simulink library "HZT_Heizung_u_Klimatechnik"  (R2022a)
settings: Solver=VariableStepAuto  StartTime=0.0  StopTime=10.0  RelTol=1e-3
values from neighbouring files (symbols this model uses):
  PAR_HZT_MaxLeistung_Heizung = 10000    [parameter_HZT.m]
  PAR_HZT_MaxLeistung_Warmwasser = 4500    [parameter_HZT.m]
  PAR_HZT_MinLeistung_Klima = -10000    [parameter_HZT.m]

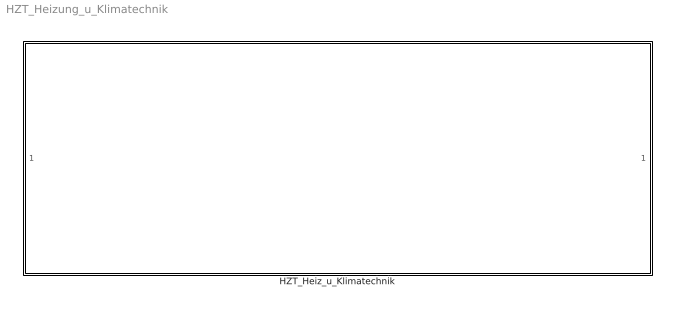
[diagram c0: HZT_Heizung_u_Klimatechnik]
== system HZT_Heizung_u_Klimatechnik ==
  HZT_Heiz_u_Klimatechnik : Subsystem

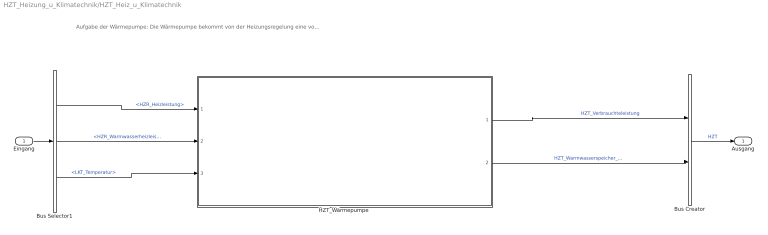
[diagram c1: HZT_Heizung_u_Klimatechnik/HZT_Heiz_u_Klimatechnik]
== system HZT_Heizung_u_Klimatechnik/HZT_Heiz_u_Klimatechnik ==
  note: Aufgabe der Wärmepumpe: Die Wärmepumpe bekommt von der Heizungsregelung eine vorgegebene Heizleistung, welche in das Haus eingespeist werden soll. Die Leistung wird dann von den Energieerzeugern genommen und umgewandelt. Das gleiche gilt für die Warmwasserheizleistung.
  Eingang : Inport
  Bus Creator : BusCreator  Inputs=2
  Bus Selector1 : BusSelector  OutputSignals=HZR.HZR_Heizleistung,HZR.HZR_Warmwasserheizleistung_Waermepumpe,LKT.LKT_Temperatur
  "HZT_Wärmepumpe " : Subsystem
  Ausgang : Outport
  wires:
  Bus Selector1/2 -> "HZT_Wärmepumpe "/2(HZR_Warmwasserheizleistung_Waermepumpe)  "<HZR_Warmwasserheizleistung_Waermepumpe>"
  "HZT_Wärmepumpe "/1(HZT_verbrauchte_Leistung) -> Bus Creator/1  "HZT_Verbrauchteleistung"
  Eingang/1 -> Bus Selector1/1
  Bus Creator/1 -> Ausgang/1  "HZT"
  "HZT_Wärmepumpe "/2(HZT_Warmwasserspeicher_verbrauchte_Leistung) -> Bus Creator/2  "HZT_Warmwasserspeicher_verbrauchte_Leistung"
  Bus Selector1/1 -> "HZT_Wärmepumpe "/1(HZR_Heizleistung)  "<HZR_Heizleistung>"
  Bus Selector1/3 -> "HZT_Wärmepumpe "/3(LKT_Temperatur)  "<LKT_Temperatur>"

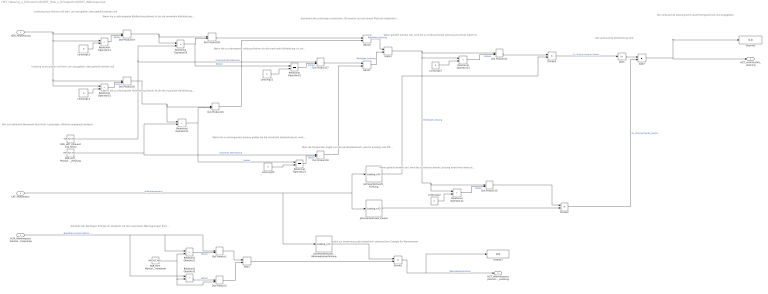
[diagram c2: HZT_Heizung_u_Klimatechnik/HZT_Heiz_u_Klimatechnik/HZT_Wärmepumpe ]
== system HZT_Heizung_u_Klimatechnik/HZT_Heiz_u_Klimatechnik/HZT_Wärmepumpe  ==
  note: Modul zur berechnung der tatsächlich verbrauchten Energie für Warmwasser
  note: Wenn die zu erbringende Kühlleistung kleiner ist als die maximale Kühlleistung, kann die angegebene Kühlleistung für die weitere Berechnung genutzt werden.
  note: Über die Temperatur ergibt sich die Jahresarbeitszahl, welche aussagt, wie Effizient die Wärmepumpe ist.
  note: Von uns definierte Maximale Heiz-/kühl- Leistungen. (Können angepasst werden)
  note: Wenn geheizt werden soll, wird die zu verbrauchende Leistung errechnet indem die Heizleistung durch die Jahresarbeitszahl geteilt wird
  note: Wenn die zu erbringende Heizleistung kleiner ist als die maximale Heizleistung, kann die angegebene Heizleistung für die weitere Berechnung genutzt werden.
  note: Leistung muss größer nulll sein, um anzugeben, dass geheizt werden soll
  note: Leistung muss kleiner nulll sein, um anzugeben, dass gekühlt werden soll
  note: Wenn die zu erbringende Leistung größer als die maximale Heizleistung ist, wird die maximale Heizleistung angenommen
  note: Wenn gekühlt werden soll, wird die zu verbrauchende Leistung errechnet indem die Kühlleistung durch die Jahresarbeitszahl geteilt wird
  note: Die verbrauchte Kühlleistung wird
  note: Kontrolle der benötigen Energie im Vergleich mit der maximalen Wärmepumpen Energie für Warmwasser.
  note: Die verbrauchte Leistung wird zusammengerechnet und angegeben
  note: Summiert alle Leistungen zusammen. (Es kommt nur aus einem Pfad ein tatsächlicher Wert, die anderen ergeben null)
  note: Wenn die zu erbringende Leistung kleiner als die maximale Kühlleistung ist, wird die maximale Kühlleistung angenommen
  HZR_Heizleistung : Inport
  HZR_Warmwasserheizleistung_Waermepumpe : Inport  Port=2
  LKT_Temperatur : Inport  Port=3
  Abs1 : Abs
  Add{1,7,10..12} (5 alike) : Sum
  Display1 : Display
  Display2 : Display
  Divide1 : Product  Inputs=/*
  Divide2 : Product  Inputs=*/
  Divide3 : Product  Inputs=*/
  Dot Product{1..2,15..21,28} (10 alike) : DotProduct
  Jahresarbeitszahl_Heizen : Lookup_n-D  NumberOfTableDimensions=1  BreakpointsForDimension1=[-20;-15;-10;-5;0;5;10;20;30]  Table=[1.5;1.7;2.05;2.4;2.7;3;3.2;3.5;3.7]  InternalRulePriority=Speed  RndMeth=Simplest
  Jahresarbeitszahl_Kühlung : Lookup_n-D  NumberOfTableDimensions=1  BreakpointsForDimension1=[20;25;30;35;40]  Table=[3.7;3.2;2.8;2.2;1.5]  InternalRulePriority=Speed  RndMeth=Simplest
  Jahresarbeitszahl_Warmwassererhitzung : Lookup_n-D  NumberOfTableDimensions=1  BreakpointsForDimension1=[-20;-15;-10;-5;0;5;10;15;20;25;30;35;40]  Table=[1.3;1.5;1.7;1.9;2.1;2.3;2.5;2.7;2.9;3.1;3.3;3.5;3.7]  InternalRulePriority=Speed  RndMeth=Simplest
  Leistung{12..15,21..22} (6 alike) : Constant  Value=0
  PAR_HZT_MaxLeistung_Heizung : Constant  Value=PAR_HZT_MaxLeistung_Heizung
  PAR_HZT_MaxLeistung_Warmwasser : Constant  Value=PAR_HZT_MaxLeistung_Warmwasser
  PAR_HZT_MinLeistung_Klima : Constant  Value=PAR_HZT_MinLeistung_Klima
  Relational Operator{1,13..14,21} (4 alike) : RelationalOperator  Operator=<  OutDataTypeStr=boolean  RndMeth=Simplest
  Relational Operator{2,12,15,20} (4 alike) : RelationalOperator  Operator=>  OutDataTypeStr=boolean  RndMeth=Simplest
  Relational Operator22 : RelationalOperator  Operator===  OutDataTypeStr=boolean  RndMeth=Simplest
  Relational Operator23 : RelationalOperator  Operator===  OutDataTypeStr=boolean  RndMeth=Simplest
  HZT_verbrauchte_Leistung : Outport
  HZT_Warmwasserspeicher_verbrauchte_Leistung : Outport  Port=2
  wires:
  Relational Operator1/1 -> Dot Product1/2  "Heizen"
  Relational Operator20/1 -> Dot Product28/2, Relational Operator22/1  "Kühlen"
  Dot Product17/1 -> Add11/1
  Leistung21/1 -> Relational Operator22/2
  PAR_HZT_MaxLeistung_Heizung/1 -> Dot Product18/1, Relational Operator21/2  "maximale Heizleistung"
  Dot Product19/1 -> Dot Product28/1, Relational Operator20/1
  Leistung14/1 -> Relational Operator15/2
  Dot Product2/1 -> Add1/2
  Divide1/1 -> HZT_Warmwasserspeicher_verbrauchte_Leistung/1, Display1/1  "Warmwasserleistung"
  Relational Operator23/1 -> Dot Product18/2  "Heizen"
  HZR_Heizleistung/1 -> Dot Product19/1, Relational Operator14/1, Dot Product20/1, Relational Operator15/1
  Dot Product1/1 -> Add1/1
  Divide3/1 -> Abs1/1  "Zu_Verbrauchende_Kühlleistung"
  PAR_HZT_MinLeistung_Klima/1 -> Dot Product17/1, Relational Operator20/2  "maximale Klimaleistung"
  LKT_Temperatur/1 -> Jahresarbeitszahl_Kühlung/1, Jahresarbeitszahl_Heizen/1, Jahresarbeitszahl_Warmwassererhitzung/1  "Außentemperatur"
  Relational Operator2/1 -> Dot Product2/1  "Heizen"
  Relational Operator21/1 -> Relational Operator23/1, Dot Product16/2  "Heizen"
  Dot Product20/1 -> Dot Product16/1, Relational Operator21/1
  Jahresarbeitszahl_Kühlung/1 -> Divide3/2
  Jahresarbeitszahl_Heizen/1 -> Divide2/2
  Dot Product16/1 -> Add10/2
  Leistung12/1 -> Relational Operator12/2
  Abs1/1 -> Add7/1
  Dot Product21/1 -> Divide3/1
  Add11/1 -> Add12/2  "Benötigte Leistung"
  Dot Product15/1 -> Divide2/1
  Leistung22/1 -> Relational Operator23/2
  PAR_HZT_MaxLeistung_Warmwasser/1 -> Relational Operator2/2, Dot Product2/2, Relational Operator1/2
  Add7/1 -> HZT_verbrauchte_Leistung/1, Display2/1
  Add10/1 -> Add12/1  "Benötigte Leistung"
  Add12/1 -> Relational Operator13/1, Relational Operator12/1, Dot Product15/1, Dot Product21/1  "Benötigte Leistung"
  Leistung15/1 -> Relational Operator13/2
  Dot Product28/1 -> Add10/1
  Jahresarbeitszahl_Warmwassererhitzung/1 -> Divide1/1
  Add1/1 -> Divide1/2
  Dot Product18/1 -> Add11/2
  HZR_Warmwasserheizleistung_Waermepumpe/1 -> Relational Operator2/1, Dot Product1/1, Relational Operator1/1  "Benötigte Leistung Warmwasser"
  Divide2/1 -> Add7/2  "Zu_Verbrauchende_Heizleistung"
  Relational Operator12/1 -> Dot Product15/2  "Heizen"
  Relational Operator22/1 -> Dot Product17/2  "Kühlen"
  Relational Operator14/1 -> Dot Product19/2  "Kühlen"
  Relational Operator13/1 -> Dot Product21/2  "Kühlen"
  Leistung13/1 -> Relational Operator14/2
  Relational Operator15/1 -> Dot Product20/2  "Heizen"
